DATA_BLOCK "DATI ENCODER"
AUTHOR : Diego_M
VERSION : 0.1


  STRUCT
   STAT0 : REAL ;
   STAT1 : REAL ;
   STAT2 : REAL ;
   STAT3 : REAL ;
   STAT4 : REAL ;
   ESPAN_ASPO : REAL ;	//ESPANSIONE ASPO
   VEL_MAX_SPIAN : REAL ;	//VELOCITA' ALTA SPIANATRICE
   STAT7 : DINT ;
   STAT8 : DINT ;
   COMP_ING : REAL ;	//COMPENETRAZIONE INGRESSO
   COMP_USC : REAL ;	//COMPENETRAZIONE USCITA
   SPIAN_JOG : REAL ;	//VELOCITA'SPIANATRICE IN JOG
   VEL_MED_SPIAN : REAL ;	//VELOCITA' MEDIA SPIANATRICE
   Tiro : REAL  := 4.000000e+008;	//Tensione nastro Kg.0-500
   LARG_COIL : REAL ;	//LARGHEZZA COIL
   STAT15 : DWORD ;
   STAT16 : DWORD ;
   NOCOMUNICAZ : INT ;
   STAT18 : DWORD ;
   STAT19 : DWORD ;
   STAT20 : DWORD ;
   STAT21 : DWORD ;
   STAT22 : DWORD ;
   STAT23 : DWORD ;
   STAT24 : DWORD ;
   STAT25 : DWORD ;
   STAT26 : DWORD ;
   STAT27 : DWORD ;
   STAT28 : DWORD ;
   STAT29 : DWORD ;
   STAT30 : DWORD ;
   STAT31 : DWORD ;
   STAT32 : DWORD ;
   STAT33 : DWORD ;
   STAT34 : DWORD ;
   STAT35 : DWORD ;
   STAT36 : DWORD ;
   STAT37 : DWORD ;
   VEL_BASSA_SPIAN : REAL ;	//VELOCITA' BASSA SPIANATRICE
   STAT40 : DWORD ;
   STAT41 : WORD ;
   STAT42 : WORD ;
   STAT43 : WORD ;
   STAT44 : WORD ;
   STAT45 : WORD ;
   STAT46 : WORD ;
   STAT47 : WORD ;
   STAT48 : WORD ;
   STAT49 : WORD ;
   STAT50 : WORD ;
   STAT52 : WORD ;
   STAT54 : WORD ;
   STAT55 : WORD ;
   STAT56 : WORD ;
   STAT57 : WORD ;
   STAT58 : WORD ;
   STAT59 : WORD ;
   STAT60 : WORD ;
   STAT61 : WORD ;
   STAT62 : WORD ;
   STAT63 : WORD ;
   STAT64 : WORD ;
   STAT65 : WORD ;
   stat66 : DWORD ;	//Corrente motore spianatrice
   STAT67 : DWORD ;
   STAT68 : DWORD ;
   STAT69 : WORD ;
   STAT70 : WORD ;
   STAT71 : WORD ;
   STAT72 : WORD ;
   STAT73 : WORD ;
   STAT74 : WORD ;
   STAT75 : WORD ;
   STAT76 : WORD ;
   STAT77 : WORD ;
   STAT78 : WORD ;
   STAT79 : WORD ;
   STAT80 : WORD ;
   STAT81 : WORD ;
   DBD242 : DWORD ;
   DBD246 : DWORD ;
   DBD250 : DWORD ;
   DBD254 : DWORD ;
   DBD258 : DWORD ;
   DBD262 : DWORD ;
   DBD266 : DWORD ;
   DBD270 : DWORD ;
   DBD274 : DWORD ;
   DBD278 : DWORD ;
   DBD282 : DWORD ;
   DBD286 : DWORD ;
   DBD290 : DWORD ;
   DBD294 : DWORD ;
   DBD298 : DWORD ;
   DBD302 : DWORD ;
   DBD306 : DWORD ;
  END_STRUCT ;
BEGIN
   STAT0 := 6.939218e-038;
   STAT1 := 5.359164e-042;
   STAT2 := 5.000000e+002;
   STAT3 := 0.000000e+000;
   STAT4 := 1.000000e+002;
   ESPAN_ASPO := 7.000000e+001;
   VEL_MAX_SPIAN := 2.000000e+001;
   STAT7 := L#10;
   STAT8 := L#1000;
   COMP_ING := 0.000000e+000;
   COMP_USC := 0.000000e+000;
   SPIAN_JOG := 1.000000e+001;
   VEL_MED_SPIAN := 1.000000e+001;
   Tiro := 0.000000e+000;
   LARG_COIL := 0.000000e+000;
   STAT15 := DW#16#34A80000;
   STAT16 := DW#16#204798;
   NOCOMUNICAZ := 0;
   STAT18 := DW#16#0;
   STAT19 := DW#16#0;
   STAT20 := DW#16#24C80000;
   STAT21 := DW#16#28F;
   STAT22 := DW#16#24E80000;
   STAT23 := DW#16#5;
   STAT24 := DW#16#13C8;
   STAT25 := DW#16#0;
   STAT26 := DW#16#24A80000;
   STAT27 := DW#16#14C80000;
   STAT28 := DW#16#14E80000;
   STAT29 := DW#16#0;
   STAT30 := DW#16#24000000;
   STAT31 := DW#16#14000000;
   STAT32 := DW#16#14000000;
   STAT33 := DW#16#15000000;
   STAT34 := DW#16#9C40;
   STAT35 := DW#16#12C;
   STAT36 := DW#16#5;
   STAT37 := DW#16#0;
   VEL_BASSA_SPIAN := 4.000000e+000;
   STAT40 := DW#16#0;
   STAT41 := W#16#0;
   STAT42 := W#16#0;
   STAT43 := W#16#0;
   STAT44 := W#16#0;
   STAT45 := W#16#0;
   STAT46 := W#16#0;
   STAT47 := W#16#0;
   STAT48 := W#16#0;
   STAT49 := W#16#0;
   STAT50 := W#16#0;
   STAT52 := W#16#0;
   STAT54 := W#16#0;
   STAT55 := W#16#0;
   STAT56 := W#16#0;
   STAT57 := W#16#0;
   STAT58 := W#16#0;
   STAT59 := W#16#0;
   STAT60 := W#16#0;
   STAT61 := W#16#0;
   STAT62 := W#16#0;
   STAT63 := W#16#0;
   STAT64 := W#16#0;
   STAT65 := W#16#0;
   stat66 := DW#16#0;
   STAT67 := DW#16#0;
   STAT68 := DW#16#0;
   STAT69 := W#16#0;
   STAT70 := W#16#0;
   STAT71 := W#16#0;
   STAT72 := W#16#0;
   STAT73 := W#16#0;
   STAT74 := W#16#0;
   STAT75 := W#16#0;
   STAT76 := W#16#0;
   STAT77 := W#16#0;
   STAT78 := W#16#0;
   STAT79 := W#16#0;
   STAT80 := W#16#0;
   STAT81 := W#16#0;
   DBD242 := DW#16#0;
   DBD246 := DW#16#0;
   DBD250 := DW#16#0;
   DBD254 := DW#16#0;
   DBD258 := DW#16#0;
   DBD262 := DW#16#0;
   DBD266 := DW#16#0;
   DBD270 := DW#16#0;
   DBD274 := DW#16#0;
   DBD278 := DW#16#0;
   DBD282 := DW#16#0;
   DBD286 := DW#16#0;
   DBD290 := DW#16#0;
   DBD294 := DW#16#0;
   DBD298 := DW#16#0;
   DBD302 := DW#16#0;
   DBD306 := DW#16#0;
END_DATA_BLOCK

